|   TEXAS INSTRUMENTS INCORPORATED
|   Standard Linear and Logic
|   IBIS Model of SN74HCT245
|   OCTAL BUS TRANSCEIVERS WITH 3-STATE OUTPUTS
|   SSOP 20-pin (DB), SOIC 20-pin (DW), P-DIP 20-pin(N), SOP 20-pin (NS),
|   TSSOP 20-pin (PW), TVSOP 20-pin (DGV), QFN 20-pin (RGY) packages.
[IBIS Ver]   3.2
[Comment Char]  |_char
[File Name]   sn74hct245.ibs
[File Rev]   1.2 | x_die
[Date]   Nov.10, 2004
[Source]   File originated at Texas Instruments, Inc.
[Notes]   The following is a sample IBIS file for the HCT245.
   - FILE REV HISTORY
   - 1.2 Re-Release IBIS file on 11/10/04
|   - All test data contained in this file are derived from
|   actual measurements.
|   - The measurement used NS packag.
|   - File created by Nobuhisa Ohtsubo, TIJ SLL Product Engineering.
[Disclaimer] Property of Texas Instruments Incorporated.  Unauthorized
   reproduction and/or distribution is strictly prohibited.
   This product is protected under copyright law.
   Created 2000, (C) Copyright 2000, Texas Instruments Inc.,
   All Rights Reserved.
   UNLESS THERE IS A SIGNED, WRITTEN AGREEMENT TO THE
   CONTRARY, TEXAS INSTRUMENTS () IS PROVIDING THE IBIS
   MODELS  AND WITHOUT ANY WARRANTY, EXPRESSED OR
   IMPLIED.  TI assumes no liability for:
   1) the accuracy of the IBIS models provided to your
   company;
   2) the proper functioning of these IBIS Models in your
   design or for any resulting applications; or
   3) infringement of patents, copyrights or intellectual
   property rights resulting from your use of these IBIS
   models.
   TI provides IBIS Models as a service to our customers.
   You and your company shall not distribute, sell or give
   these models to anyone else without prior written
   permission from TI.
   TI reserves the right to make changes to our products or
   to discontinue any semiconductor product or service
   without notice, and advises our customers to obtain the
   latest version of relevant information to verify, before
   placing orders, that the information being relied on is
   current.
   Please be aware that your receipt and use of the IBIS
   information provided shall serve as acceptance of these
   terms and conditions.  If you do not accept these terms,
   you should return or destroy the IBIS models and any
   other accompanying information immediately.
|   Component HCT245_DB
[Component]   HCT245_DB
[Manufacturer]  Texas Instruments, Inc.
[Package]
|   typ   min   max
R_pkg   0.040   0.035   0.051
L_pkg   3.495nH   3.035nH   4.314nH
C_pkg   0.420pF   0.346pF   0.502pF
[Pin]   signal_name   model_name   R_pin   L_pin   C_pin
1   DIR   HCT245_DIR   0.049   4.310nH   0.502pF
2   A1   HCT245_IO   0.048   3.903nH   0.487pF
3   A2   HCT245_IO   0.035   3.189nH   0.396pF
4   A3   HCT245_IO   0.035   3.036nH   0.347pF
5   A4   HCT245_IO   0.035   3.035nH   0.367pF
6   A5   HCT245_IO   0.035   3.035nH   0.367pF
7   A6   HCT245_IO   0.035   3.036nH   0.347pF
8   A7   HCT245_IO   0.035   3.189nH   0.397pF
9   A8   HCT245_IO   0.047   3.899nH   0.488pF
10   GND   GND   0.051   4.314nH   0.500pF
11   B8   HCT245_IO   0.051   4.314nH   0.500pF
12   B7   HCT245_IO   0.047   3.899nH   0.488pF
13   B6   HCT245_IO   0.035   3.189nH   0.397pF
14   B5   HCT245_IO   0.035   3.036nH   0.346pF
15   B4   HCT245_IO   0.035   3.035nH   0.367pF
16   B3   HCT245_IO   0.035   3.035nH   0.367pF
17   B2   HCT245_IO   0.035   3.036nH   0.346pF
18   B1   HCT245_IO   0.035   3.189nH   0.397pF
19   NOE   HCT245_NOE   0.047   3.899nH   0.488pF
20   VCC   POWER   0.051   4.314nH   0.502pF
|   Component HCT245_DW
[Component]   HCT245_DW
[Manufacturer]  Texas Instruments, Inc.
[Package]
|   typ   min   max
R_pkg   0.038   0.033   0.045
L_pkg   5.012nH   4.110nH   6.349nH
C_pkg   0.717pF   0.530pF   0.868pF
[Pin]   signal_name   model_name   R_pin   L_pin   C_pin
1   DIR   HCT245_DIR   0.058   5.115nH   0.725pF
2   A1   HCT245_IO   0.053   4.591nH   0.724pF
3   A2   HCT245_IO   0.049   3.754nH   0.572pF
4   A3   HCT245_IO   0.029   2.549nH   0.388pF
5   A4   HCT245_IO   0.031   2.317nH   0.316pF
6   A5   HCT245_IO   0.031   2.317nH   0.316pF
7   A6   HCT245_IO   0.029   2.556nH   0.399pF
8   A7   HCT245_IO   0.049   3.754nH   0.579pF
9   A8   HCT245_IO   0.053   4.591nH   0.724pF
10   GND   GND   0.058   5.115nH   0.725pF
11   B8   HCT245_IO   0.058   5.115nH   0.725pF
12   B7   HCT245_IO   0.053   4.591nH   0.724pF
13   B6   HCT245_IO   0.049   3.754nH   0.579pF
14   B5   HCT245_IO   0.029   2.557nH   0.399pF
15   B4   HCT245_IO   0.031   2.317nH   0.316pF
16   B3   HCT245_IO   0.031   2.317nH   0.316pF
17   B2   HCT245_IO   0.029   2.557nH   0.399pF
18   B1   HCT245_IO   0.049   3.754nH   0.579pF
19   NOE   HCT245_NOE   0.053   4.591nH   0.724pF
20   VCC   POWER   0.058   5.115nH   0.725pF
| Component HCT245_N 20-pin PDIP
[Component]   HCT245_N
[Manufacturer]   Texas Instruments, Inc.
[Package]
|   typ   min   max
R_pkg   4.300e-02   3.800e-02   5.000e-02
L_pkg   7.384e-09   4.680e-09   1.032e-08
C_pkg   5.100e-13   2.310e-13   8.210e-13
[Pin]   signal_name   model_name   R_pin   L_pin   C_pin
1   DIR   HCT245_DIR   4.200e-02   9.427e-09   8.100e-13
2   A1   HCT245_IO   4.600e-02   8.544e-09   4.560e-13
3   A2   HCT245_IO   4.800e-02   7.163e-09   4.350e-13
4   A3   HCT245_IO   4.000e-02   4.825e-09   2.610e-13
5   A4   HCT245_IO   4.000e-02   5.284e-09   6.480e-13
6   A5   HCT245_IO   4.000e-02   4.686e-09   2.320e-13
7   A6   HCT245_IO   4.000e-02   6.359e-09   4.890e-13
8   A7   HCT245_IO   3.800e-02   7.982e-09   4.750e-13
9   A8   HCT245_IO   4.300e-02   9.403e-09   4.750e-13
10   GND   GND   5.000e-02   1.032e-08   8.050e-13
11   B8   HCT245_IO   5.000e-02   1.028e-08   8.100e-13
12   B7   HCT245_IO   4.300e-02   9.383e-09   4.770e-13
13   B6   HCT245_IO   3.800e-02   7.978e-09   4.760e-13
14   B5   HCT245_IO   4.000e-02   6.302e-09   4.920e-13
15   B4   HCT245_IO   4.000e-02   4.680e-09   2.310e-13
16   B3   HCT245_IO   4.000e-02   5.284e-09   6.480e-13
17   B2   HCT245_IO   4.000e-02   4.822e-09   2.610e-13
18   B1   HCT245_IO   4.700e-02   7.118e-09   4.390e-13
19   NOE   HCT245_NOE   4.600e-02   8.492e-09   4.610e-13
20   VCC   POWER   4.300e-02   9.348e-09   8.210e-13
|   Component HCT245_NS
[Component]   HCT245_NS
[Manufacturer]  Texas Instruments, Inc.
[Package]
|   typ   min   max
R_pkg   0.044   0.029   0.058
L_pkg   3.666nH   2.317nH   5.115nH
C_pkg   0.548pF   0.316pF   0.725pF
[Pin]   signal_name   model_name   R_pin   L_pin   C_pin
1   DIR   HCT245_DIR   0.058   5.115nH   0.725pF
2   A1   HCT245_IO   0.053   4.591nH   0.724pF
3   A2   HCT245_IO   0.049   3.754nH   0.572pF
4   A3   HCT245_IO   0.029   2.549nH   0.388pF
5   A4   HCT245_IO   0.031   2.317nH   0.316pF
6   A5   HCT245_IO   0.031   2.317nH   0.316pF
7   A6   HCT245_IO   0.029   2.556nH   0.399pF
8   A7   HCT245_IO   0.049   3.754nH   0.579pF
9   A8   HCT245_IO   0.053   4.591nH   0.724pF
10   GND   GND   0.058   5.115nH   0.725pF
11   B8   HCT245_IO   0.058   5.115nH   0.725pF
12   B7   HCT245_IO   0.053   4.591nH   0.724pF
13   B6   HCT245_IO   0.049   3.754nH   0.579pF
14   B5   HCT245_IO   0.029   2.557nH   0.399pF
15   B4   HCT245_IO   0.031   2.317nH   0.316pF
16   B3   HCT245_IO   0.031   2.317nH   0.316pF
17   B2   HCT245_IO   0.029   2.557nH   0.399pF
18   B1   HCT245_IO   0.049   3.754nH   0.579pF
19   NOE   HCT245_NOE   0.053   4.591nH   0.724pF
20   VCC   POWER   0.058   5.115nH   0.725pF
|   Component HCT245_PW
[Component]   HCT245_PW
[Manufacturer]  Texas Instruments, Inc.
[Package]
|   typ   min   max
R_pkg   0.035   0.024   0.047
L_pkg   2.399nH   1.710nH   3.250nH
C_pkg   0.284pF   0.166pF   0.418pF
[Pin]   signal_name   model_name   R_pin   L_pin   C_pin
1   DIR   HCT245_DIR   0.041   3.102nH   0.410pF
2   A1   HCT245_IO   0.040   2.777nH   0.363pF
3   A2   HCT245_IO   0.029   2.194nH   0.260pF
4   A3   HCT245_IO   0.025   1.710nH   0.166pF
5   A4   HCT245_IO   0.025   1.740nH   0.191pF
6   A5   HCT245_IO   0.024   1.763nH   0.193pF
7   A6   HCT245_IO   0.024   1.817nH   0.174pF
8   A7   HCT245_IO   0.028   2.256nH   0.265pF
9   A8   HCT245_IO   0.045   2.887nH   0.368pF
10   GND   GND   0.047   3.250nH   0.417pF
11   B8   HCT245_IO   0.046   3.244nH   0.418pF
12   B7   HCT245_IO   0.046   2.961nH   0.375pF
13   B6   HCT245_IO   0.033   2.334nH   0.268pF
14   B5   HCT245_IO   0.029   1.915nH   0.179pF
15   B4   HCT245_IO   0.031   1.934nH   0.203pF
16   B3   HCT245_IO   0.032   1.917nH   0.201pF
17   B2   HCT245_IO   0.030   1.833nH   0.173pF
18   B1   HCT245_IO   0.036   2.324nH   0.268pF
19   NOE   HCT245_NOE   0.042   2.869nH   0.372pF
20   VCC   POWER   0.042   3.160nH   0.414pF
|   Component HCT245_DGV
[Component]   HCT245_DGV
[Manufacturer]  Texas Instruments, Inc.
[Package]
|   typ   min   max
R_pkg   4.400e-02   3.800e-02   4.800e-02
L_pkg   2.561e-09   2.236e-09   2.961e-09
C_pkg   3.420e-13   2.640e-13   4.460e-13
[Pin]   signal_name   model_name   R_pin   L_pin   C_pin
1   DIR   HCT245_DIR   4.400e-02   2.935e-09   4.170e-13
2   A1   HCT245_IO   4.200e-02   2.869e-09   4.460e-13
3   A2   HCT245_IO   4.300e-02   2.399e-09   3.160e-13
4   A3   HCT245_IO   4.400e-02   2.236e-09   2.650e-13
5   A4   HCT245_IO   4.600e-02   2.278e-09   2.640e-13
6   A5   HCT245_IO   4.500e-02   2.274e-09   2.640e-13
7   A6   HCT245_IO   4.400e-02   2.285e-09   2.690e-13
8   A7   HCT245_IO   4.300e-02   2.452e-09   3.200e-13
9   A8   HCT245_IO   4.400e-02   2.900e-09   4.460e-13
10   GND   GND   4.400e-02   2.961e-09   4.180e-13
11   B8   HCT245_IO   4.500e-02   2.954e-09   4.180e-13
12   B7   HCT245_IO   4.200e-02   2.847e-09   4.430e-13
13   B6   HCT245_IO   4.500e-02   2.453e-09   3.190e-13
14   B5   HCT245_IO   4.500e-02   2.297e-09   2.690e-13
15   B4   HCT245_IO   4.800e-02   2.334e-09   2.680e-13
16   B3   HCT245_IO   4.800e-02   2.335e-09   2.670e-13
17   B2   HCT245_IO   4.600e-02   2.299e-09   2.680e-13
18   B1   HCT245_IO   4.600e-02   2.457e-09   3.200e-13
19   NOE   HCT245_NOE   4.300e-02   2.848e-09   4.410e-13
20   VCC   POWER   3.800e-02   2.812e-09   4.080e-13
|   Component HCT245_RGY
[Component]   HCT245_RGY
[Manufacturer]   Texas Instruments, Inc.
[Package]
|   typ   min   max
R_pkg   0.046   0.035   0.058
L_pkg   1.131nH   0.880nH   1.396nH
C_pkg   0.165pF   0.142pF   0.175pF
[Pin]   signal_name   model_name   R_pin   L_pin   C_pin
1   DIR   HCT245_DIR   0.053   1.289nH   0.142pF
2   A1   HCT245_IO   0.058   1.386nH   0.172pF
3   A2   HCT245_IO   0.046   1.111nH   0.173pF
4   A3   HCT245_IO   0.039   0.965nH   0.161pF
5   A4   HCT245_IO   0.035   0.881nH   0.165pF
6   A5   HCT245_IO   0.035   0.880nH   0.165pF
7   A6   HCT245_IO   0.039   0.961nH   0.161pF
8   A7   HCT245_IO   0.045   1.105nH   0.172pF
9   A8   HCT245_IO   0.058   1.386nH   0.172pF
10   GND   GND   0.056   1.352nH   0.159pF
11   B8   HCT245_IO   0.053   1.287nH   0.155pF
12   B7   HCT245_IO   0.058   1.396nH   0.172pF
13   B6   HCT245_IO   0.047   1.129nH   0.175pF
14   B5   HCT245_IO   0.040   0.976nH   0.164pF
15   B4   HCT245_IO   0.035   0.884nH   0.169pF
16   B3   HCT245_IO   0.035   0.881nH   0.168pF
17   B2   HCT245_IO   0.039   0.967nH   0.162pF
18   B1   HCT245_IO   0.046   1.118nH   0.174pF
19   NOE   HCT245_NOE   0.058   1.396nH   0.175pF
20   VCC   POWER   0.052   1.276nH   0.144pF
| Models and submodels in the file (3): HCT245_DIR (Input), HCT245_NOE (Input), HCT245_IO (I/O)
